[IBIS Ver] 2.1
[File Name] sprm016.ibs
[File Rev] 0.1
[Date] January 31, 2001
[Source] IBIS Model Generated from PACED 4.40B
[Disclaimer]   Please be aware that in the absence of a written agreement
|   Texas Instruments(TI) assumes no liability for:
|   (1) The accuracy of the IBIS models provided to your company
|   (2) The proper functioning of these Models in your design
|   or for any resulting applications; or
|   (3)Infringement of patents, copyrights or intellectual
|   property rights resulting from your use of these models.
|   TI provides IBIS Models as a service to our customers and
|   therefore reserves the right to limit distribution of the
|   Models.
[Copyright]   Property of Texas Instruments Incorporated.
|   Unauthorized reproduction and/or distribution is strictly.
|   prohibited.
|   This product is protected under copyright law and trade
|   secret law as an unpublished work.
|   Created 1999,(C) Copyright 1999-2000,
|   Texas Instruments Incorporated., All Rights Reserved.
|   These commodities are under the U.S.
|   Government distribution license control. As such,they are
|   not to be re-exported without the prior approval of the U.S.
|   Department of Commerce.
[Component]   c6205_GHK
[Manufacturer]  Texas Instruments
[Package]
|Variable Typ   Min   Max
R_pkg   0.1434   0.02894  0.4105
L_pkg   3.05E-09 6.40E-10 7.88E-09
C_pkg   3.35E-13 7.50E-14 6.48E-13
[Pin]signal_name   model_name   R_pin   L_pin   C_pin
J3   CLKI   IDH041   0.1101  2.47E-09  3.01E-13
T18  CLKOUT1   OUH831   0.1985  4.10E-09 4.91E-13
T19  CLKOUT2   OUH831   0.2544  5.11E-09  5.43E-13
L3   CLKMD0   IDH041   0.1055  2.45E-09  3.10E-13
E17  TMS   IDH041_PS1001   0.1354  3.05E-09  3.66E-13
D19  TDO   OUH831   0.2574  5.16E-09  5.23E-13
D18  TDI   IDH041_PS1001   0.1932  4.07E-09  4.96E-13
D17  TCLK   IDH041   0.1482  3.25E-09  3.41E-13
C19  TRSTz   IDH041_PE1001   0.2607  5.21E-09  5.28E-13
E18  EMU1   IDH041_OUH831_PE1001 0.1789  3.81E-09  3.97E-13
F15  EMU0   IDH041_OUH831_PE1001 0.1035  2.46E-09  2.90E-13
C3   RESETz   UIS341   0.1710  3.78E-09  4.26E-13
A8   NMI   IDH041   0.2131  4.34E-09  4.71E-13
B15  EXT_INT7   IDH041_OUI431   0.1895  3.95E-09  4.46E-13
C15  EXT_INT6   IDH041   0.1339  3.04E-09  3.93E-13
A16  EXT_INT5   IDH041_OUI431   0.2763  5.46E-09  5.42E-13
B16  EXT_INT4   IDH041_OUI431   0.2029  4.24E-09  5.22E-13
A15  IACK   IDH041_OUI431   0.2266  4.58E-09  4.93E-13
F12  INUM3   IDH041_OUI431   0.1453  3.18E-09  3.33E-13
A14  INUM2   IDH041_OUI431   0.2148  4.40E-09  4.13E-13
B14  INUM1   IDH041_OUI431   0.1873  3.97E-09  4.24E-13
C14  INUM0   IDH041_OUI431   0.1324  2.96E-09  3.74E-13
B18  PD   OUI431   0.2409  4.93E-09  4.92E-13
W5   PCLK   UBS032   0.2255  4.60E-09  4.72E-13
D2   AD31   UBS032   0.1921  4.04E-09  4.92E-13
E3   AD30   UBS032   0.1333  3.05E-09  3.91E-13
E2   AD29   UBS032   0.1800  3.72E-09  4.33E-13
E1   AD28   UBS032   0.2395  4.83E-09  4.92E-13
F3   AD27   UBS032   0.1338  2.94E-09  3.71E-13
F5   AD26   UBS032   0.1838  3.81E-09  3.82E-13
F1   AD25   UBS032   0.2248  4.71E-09  5.00E-13
G3   AD24   UBS032   0.1140  2.62E-09  3.18E-13
H3   AD23   UBS032   0.1463  3.46E-09  4.23E-13
H2   AD22   UBS032   0.1503  3.21E-09  3.80E-13
J1   AD21   UBS032   0.1940  3.89E-09  4.53E-13
H1   AD20   UBS032   0.1860  3.78E-09  4.39E-13
M2   AD19   UBS032   0.1720  3.67E-09  4.32E-13
M1   AD18   UBS032   0.2149  4.34E-09  4.42E-13
N2   AD17   UBS032   0.1724  3.59E-09  3.88E-13
N1   AD16   UBS032   0.2119  4.29E-09  4.52E-13
T1   AD15   UBS032   0.2610  5.31E-09  4.82E-13
V2   AD14   UBS032   0.2390  5.00E-09  3.46E-13
U2   AD13   UBS032   0.2107  4.38E-09  4.60E-13
U1   AD12   UBS032   0.2650  5.33E-09  5.17E-13
W3   AD11   UBS032   0.2567  5.19E-09  6.00E-13
W2   AD10   UBS032   0.2737  5.59E-09  4.23E-13
V1   AD09   UBS032   0.2686  5.41E-09  5.50E-13
U4   AD08   UBS032   0.1485  3.29E-09  3.58E-13
W4   AD07   UBS032   0.2611  5.26E-09  5.19E-13
U5   AD06   UBS032   0.1338  3.01E-09  3.48E-13
V5   AD05   UBS032   0.2029  4.26E-09  4.64E-13
U6   AD04   UBS032   0.1332  2.98E-09  3.73E-13
V6   AD03   UBS032   0.1884  3.99E-09  4.39E-13
V3   AD02   UBS032   0.4105  7.88E-09  6.48E-13
W6   AD01   UBS032   0.1908  4.21E-09  4.75E-13
U7   AD00   UBS032   0.1426  2.90E-09  2.91E-13
G2   PCBE3z   UBS032   0.1592  3.34E-09  4.03E-13
M3   PCBE2z   UBS032   0.1133  2.60E-09  3.33E-13
T2   PCBE1z   UBS032   0.1974  4.20E-09  4.95E-13
V4   PCBE0z   UBS032   0.1905  4.07E-09  4.95E-13
C1   PINTAz   UBS032   0.2578  5.11E-09  5.38E-13
F2   PREQz   UBS032   0.1926  4.04E-09  4.36E-13
P5   PSERRz   UBS032   0.1361  3.08E-09  3.65E-13
P2   PPERRz   UBS032   0.1769  3.73E-09  4.12E-13
C2   PRSTz   UBS032   0.2541  5.14E-09  4.77E-13
R2   PDEVSELz   UBS032   0.1896  3.97E-09  4.09E-13
D1   PGNTz   UBS032   0.2556  5.08E-09  5.16E-13
N5   PFRAMEz   UBS032   0.1256  2.94E-09  3.22E-13
P1   PIRDYz   UBS032   0.2157  4.38E-09  4.45E-13
T3   PPAR   UBS032   0.1679  3.68E-09  4.09E-13
H5   PIDSEL   UBS032   0.08213 1.84E-09  2.15E-13
R1   PSTOPz   UBS032   0.2271  4.59E-09  4.80E-13
N3   PTRDYz   UBS032   0.1271  2.84E-09  3.28E-13
C17  XSP_CLK   OUI431   0.2048  4.32E-09  3.51E-13
C18  XSP_DI   IDH041_PE1001   0.2043  4.29E-09  4.43E-13
B19  XSP_DO   OUI431   0.2715  5.41E-09  4.39E-13
C11  XSP_CS   OUI431   0.1094  2.50E-09  2.87E-13
B1   3.3VauxDET   UIS327   0.2681  5.53E-09  3.67E-13
D3   PME   UOS292   0.1467  3.29E-09  2.87E-13
A2   PWR_WKPz   UIS328   0.2754  5.34E-09  4.82E-13
V18  CE3z   OUH831   0.2370  5.02E-09  3.93E-13
U17  CE2z   OUH831   0.1724  3.57E-09  3.42E-13
W18  CE1z   OUH831   0.2476  5.05E-09  5.06E-13
V17  CE0z   OUH831   0.1909  4.20E-09  4.88E-13
U16  BE3z   OUH831   0.1649  3.42E-09  3.54E-13
W17  BE2z   OUH831   0.2615  5.23E-09  5.15E-13
V16  BE1z   OUH831   0.1724  3.90E-09  5.12E-13
W16  BE0z   OUH831   0.2579  5.19E-09  5.10E-13
V7   EA21   IDH041_OUH831_PE1001 0.1531  3.29E-09  3.91E-13
W7   EA20   IDH041_OUH831_PE1001 0.1864  4.02E-09  4.50E-13
U8   EA19   IDH041_OUH831_PE1001 0.1484  2.96E-09  3.34E-13
V8   EA18   IDH041_OUH831_PE1001 0.1394  3.07E-09  3.69E-13
W8   EA17   IDH041_OUH831   0.1884  3.85E-09  4.41E-13
W9   EA16   IDH041_OUH831   0.1996  3.96E-09  4.52E-13
V9   EA15   IDH041_OUH831   0.1199  2.98E-09  4.19E-13
U9   EA14   IDH041_OUH831   0.1281  2.79E-09  3.42E-13
W10  EA13   IDH041_OUH831   0.1780  3.69E-09  4.20E-13
V10  EA12   IDH041_OUH831   0.1508  3.45E-09  4.37E-13
U10  EA11   IDH041_OUH831   0.1261  2.64E-09  2.82E-13
W11  EA10   IDH041_OUH831   0.1922  3.96E-09  4.19E-13
V11  EA09   IDH041_OUH831   0.1339  3.10E-09  3.94E-13
U11  EA08   IDH041_OUH831   0.1372  2.85E-09  2.90E-13
R11  EA07   IDH041_OUH831   0.1198  2.76E-09  3.21E-13
W12  EA06   IDH041_OUH831   0.1902  4.20E-09  4.38E-13
U12  EA05   IDH041_OUH831   0.1394  2.87E-09  2.61E-13
R12  EA04   IDH041_OUH831   0.1467  3.23E-09  3.38E-13
W13  EA03   IDH041_OUH831   0.2096  4.29E-09  4.18E-13
V13  EA02   IDH041_OUH831   0.1865  3.98E-09  4.29E-13
F14  ED31   IDH041_OUH831_PE1001 0.1489  3.32E-09  3.27E-13
E19  ED30   IDH041_OUH831_PE1001 0.2238  4.57E-09  4.48E-13
F17  ED29   IDH041_OUH831_PE1001 0.1300  2.92E-09  3.47E-13
G15  ED28   IDH041_OUH831_PE1001 0.1202  2.80E-09  3.13E-13
F18  ED27   IDH041_OUH831_PE1001 0.1754  3.69E-09  4.17E-13
F19  ED26   IDH041_OUH831_PE1001 0.2339  4.75E-09  4.73E-13
G17  ED25   IDH041_OUH831_PE1001 0.1327  2.99E-09  3.60E-13
G18  ED24   IDH041_OUH831_PE1001 0.1662  3.50E-09  4.36E-13
G19  ED23   IDH041_OUH831_PE1001 0.2370  4.76E-09  4.92E-13
H17  ED22   IDH041_OUH831_PE1001 0.1120  2.57E-09  3.19E-13
H18  ED21   IDH041_OUH831_PE1001 0.1399  3.09E-09  4.00E-13
H19  ED20   IDH041_OUH831_PE1001 0.2134  4.33E-09  4.49E-13
J18  ED19   IDH041_OUH831_PE1001 0.1406  3.10E-09  3.76E-13
J19  ED18   IDH041_OUH831_PE1001 0.2079  4.26E-09  4.44E-13
K15  ED17   IDH041_OUH831_PE1001 0.1163  2.69E-09  2.97E-13
K17  ED16   IDH041_OUH831_PE1001 0.1005  2.35E-09  2.91E-13
K18  ED15   IDH041_OUH831_PE1001 0.1397  3.03E-09  3.80E-13
K19  ED14   IDH041_OUH831_PE1001 0.2054  4.18E-09  4.45E-13
L17  ED13   IDH041_OUH831_PE1001 0.1093  2.45E-09  3.35E-13
L18  ED12   IDH041_OUH831_PE1001 0.1494  3.24E-09  3.82E-13
L19  ED11   IDH041_OUH831_PE1001 0.1918  3.85E-09  4.34E-13
M19  ED10   IDH041_OUH831_PE1001 0.1885  3.83E-09  4.40E-13
M18  ED09   IDH041_OUH831_PE1001 0.1501  3.20E-09  3.72E-13
M17  ED08   IDH041_OUH831_PE1001 0.1065  2.48E-09  3.04E-13
N19  ED07   IDH041_OUH831_PE1001 0.2102  4.30E-09  4.13E-13
P19  ED06   IDH041_OUH831_PE1001 0.2136  4.39E-09  4.09E-13
N15  ED05   IDH041_OUH831_PE1001 0.1008  2.37E-09  2.76E-13
P18  ED04   IDH041_OUH831_PE1001 0.1858  3.93E-09  4.31E-13
P17  ED03   IDH041_OUH831_PE1001 0.1292  2.90E-09  3.71E-13
R19  ED02   IDH041_OUH831_PE1001 0.2234  4.52E-09  4.84E-13
R18  ED01   IDH041_OUH831_PE1001 0.1867  3.88E-09  4.43E-13
R17  ED00   IDH041_OUH831_PE1001 0.1397  3.06E-09  3.41E-13
U14  AREz   OUH831   0.1518  3.09E-09  3.14E-13
W14  AOEz   OUH831   0.1814  3.91E-09  4.78E-13
V14  AWEz   OUH831   0.1593  3.43E-09  4.15E-13
W15  ARDY   IDH041_PE1001   0.2050  4.44E-09  5.04E-13
U19  SDA10   OUH831   0.2594  5.18E-09  5.42E-13
V19  SDCASz_SSADSz OUH831   0.2540  5.12E-09  3.57E-13
U18  SDRASz_SSOEz  OUH831   0.2248  4.52E-09  4.90E-13
T17  SDWEz_SSWEz   OUH831   0.1569  3.44E-09  4.35E-13
P14  HOLDz   IDH041   0.1487  3.26E-09  3.48E-13
V15  HOLDAz   OUH831   0.1805  3.81E-09  4.44E-13
A5   TOUT1   OUI431   0.2418  4.87E-09  5.09E-13
B5   TIN1   IDH041_PE1001   0.1890  3.97E-09  4.27E-13
E5   TOUT0   OUI431   0.1692  3.73E-09  3.69E-13
C5   TIN0   IDH041   0.1450  3.21E-09  4.09E-13
A17  DMAC3   IDH041_OUI431_PE1001 0.2417  4.83E-09  5.16E-13
B17  DMAC2   OUI431   0.2267  4.62E-09  5.00E-13
C16  DMAC1   IDH041_OUI431_PE1001 0.1297  2.95E-09  3.65E-13
A18  DMAC0   OUI431   0.2741  5.51E-09  5.50E-13
A12  CLKS0   IDH041_PE1001   0.04461 9.91E-10  1.26E-13
B9   CLKR0   IDH041_OUI431_PE1001 0.1751  3.66E-09  4.10E-13
C9   CLKX0   IDH041_OUI431_PE1001 0.1079  2.53E-09  3.39E-13
A10  DR0   IDH041_PE1001   0.2076  4.25E-09  4.24E-13
B10  DX0   OUI431   0.1686  3.56E-09  4.22E-13
E10  FSR0   IDH041_OUI431_PE1001 0.08092 1.98E-09  2.52E-13
A9   FSX0   IDH041_OUI431_PE1001 0.2137  4.33E-09  4.47E-13
C6   CLKS1   IDH041_PE1001   0.1440  3.22E-09  3.85E-13
B6   CLKR1   IDH041_OUI431_PE1001 0.1826  3.88E-09  4.53E-13
E6   CLKX1   IDH041_OUI431_PE1001 0.1444  3.20E-09  3.35E-13
A7   DR1   IDH041_PE1001   0.2246  4.58E-09  4.86E-13
B7   DX1   OUI431   0.1866  3.91E-09  4.61E-13
C7   FSR1   IDH041_OUI431_PE1001 0.1311  2.99E-09  3.85E-13
A6   FSX1   IDH041_OUI431_PE1001 0.2456  4.92E-09  5.03E-13
| End of package information
[Component]   IDH041
[Manufacturer]   Texas Instruments
[Package]
|   typ   min   max
R_pkg   0   0   0
L_pkg   0   0   0
C_pkg   0   0   0
[Pin]   signal_name   model_name   R_pin   L_pin   C_pin
   1   A   IDH041   0   0   0
[Component]   OUH831
[Manufacturer]   Texas Instruments
[Package]
|   typ   min   max
R_pkg   0   0   0
L_pkg   0   0   0
C_pkg   0   0   0
[Pin]   signal_name   model_name   R_pin   L_pin   C_pin
   1   Y   OUH831   0   0   0
[Component]   UIS327
[Manufacturer]   Texas Instruments
[Package]
|   typ   min   max
R_pkg   0   0   0
L_pkg   0   0   0
C_pkg   0   0   0
[Pin]   signal_name   model_name   R_pin   L_pin   C_pin
   1   A   UIS327   0   0   0
[Component]   OUI431
[Manufacturer]   Texas Instruments
[Package]
|   typ   min   max
R_pkg   0   0   0
L_pkg   0   0   0
C_pkg   0   0   0
[Pin]   signal_name   model_name   R_pin   L_pin   C_pin
   1   Y   OUI431   0   0   0
[Component]   UBS032
[Manufacturer]   Texas Instruments
[Package]
|   typ   min   max
R_pkg   0   0   0
L_pkg   0   0   0
C_pkg   0   0   0
[Pin]   signal_name   model_name   R_pin   L_pin   C_pin
   1   Y2   UBS032   0   0   0
[Component]   IDH041_PE1001
[Manufacturer]   Texas Instruments
[Package]
|   typ   min   max
R_pkg   0   0   0
L_pkg   0   0   0
C_pkg   0   0   0
[Pin]   signal_name   model_name   R_pin   L_pin   C_pin
   1   A   IDH041_PE1001   0   0   0
[Component]   IDH041_OUH831_PE1001
[Manufacturer]   Texas Instruments
[Package]
|   typ   min   max
R_pkg   0   0   0
L_pkg   0   0   0
C_pkg   0   0   0
[Pin]   signal_name   model_name   R_pin   L_pin   C_pin
   1   Y   IDH041_OUH831_PE1001   0   0   0
[Component]   IDH041_OUI431
[Manufacturer]   Texas Instruments
[Package]
|   typ   min   max
R_pkg   0   0   0
L_pkg   0   0   0
C_pkg   0   0   0
[Pin]   signal_name   model_name   R_pin   L_pin   C_pin
   1   Y   IDH041_OUI431   0   0   0
[Component]   UIS328
[Manufacturer]   Texas Instruments
[Package]
|   typ   min   max
R_pkg   0   0   0
L_pkg   0   0   0
C_pkg   0   0   0
[Pin]   signal_name   model_name   R_pin   L_pin   C_pin
   1   ZRINGDET   UIS328   0   0   0
[Component]   UIS341
[Manufacturer]   Texas Instruments
[Package]
|   typ   min   max
R_pkg   0   0   0
L_pkg   0   0   0
C_pkg   0   0   0
[Pin]   signal_name   model_name   R_pin   L_pin   C_pin
   1   A   UIS341   0   0   0
[Component]   IDH041_OUH831
[Manufacturer]   Texas Instruments
[Package]
|   typ   min   max
R_pkg   0   0   0
L_pkg   0   0   0
C_pkg   0   0   0
[Pin]   signal_name   model_name   R_pin   L_pin   C_pin
   1   Y   IDH041_OUH831   0   0   0
[Component]   IDH041_PS1001
[Manufacturer]   Texas Instruments
[Package]
|   typ   min   max
R_pkg   0   0   0
L_pkg   0   0   0
C_pkg   0   0   0
[Pin]   signal_name   model_name   R_pin   L_pin   C_pin
   1   A   IDH041_PS1001   0   0   0
[Component]   IDH041_OUI431_PE1001
[Manufacturer]   Texas Instruments
[Package]
|   typ   min   max
R_pkg   0   0   0
L_pkg   0   0   0
C_pkg   0   0   0
[Pin]   signal_name   model_name   R_pin   L_pin   C_pin
   1   Y   IDH041_OUI431_PE1001   0   0   0
[Component]   UOS292
[Manufacturer]   Texas Instruments
[Package]
|   typ   min   max
R_pkg   0   0   0
L_pkg   0   0   0
C_pkg   0   0   0
[Pin]   signal_name   model_name   R_pin   L_pin   C_pin
   1   PME   UOS292   0   0   0
| Models and submodels in the file (14): IDH041 (Input), OUH831 (3-state), UIS327 (Input), OUI431 (3-state), UBS032 (I/O), IDH041_PE1001 (Input), IDH041_OUH831_PE1001 (I/O), IDH041_OUI431 (I/O), UIS328 (Input), UIS341 (Input), IDH041_OUH831 (I/O), IDH041_PS1001 (Input), IDH041_OUI431_PE1001 (I/O), UOS292 (Output)
